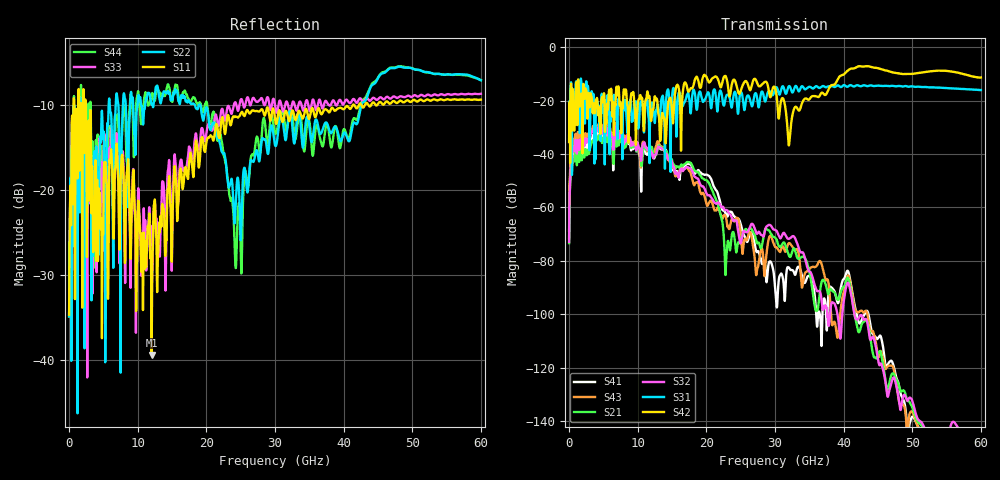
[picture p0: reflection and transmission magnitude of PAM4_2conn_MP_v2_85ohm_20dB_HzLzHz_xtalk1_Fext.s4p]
! Info: Touchstone file created by Circ.  Input file=FAB50GbE_2conn_Midplane_Examax_Topo2_v2_85ohm_20dB_HzLzHz.circ
# Hz S RI R 50
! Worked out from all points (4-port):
!   6000 points, 10 MHz to 60 GHz, reference 50 ohm
!   strongest paths, dB at 10 MHz, 15.01 GHz, 30.01 GHz, 45.01 GHz, 60 GHz:
!     S42: -35.5, -24.0, -15.3, -7.9, -11.4
!     S31: -35.4, -18.5, -15.8, -14.4, -16.1
!     S32: -72.9, -43.2, -68.4, -116.9, -151.1
!     S21: -73.4, -42.3, -71.3, -115.0, -146.2
!     S43: -71.5, -44.6, -74.7, -115.5, -158.6
!     S41: -68.7, -43.4, -90.3, -109.0, -158.7
!   lowest |S11| = -39.5 dB at 12.03 GHz (marker M1), VSWR 1.02, Z = 50.8 + j0.663 ohm
!   |S11| at or under -10 dB: start of sweep to 664.7 MHz; 2.422 GHz to 41.34 GHz (38.91 GHz wide, 178 % of centre); 41.56 GHz to 42.2 GHz (636.6 MHz wide, 1.52 % of centre)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
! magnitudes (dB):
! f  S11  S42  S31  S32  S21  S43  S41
! 10 MHz  -34.7  -35.5  -35.4  -72.9  -73.4  -71.5  -68.7
! 1.14 GHz  -12.1  -15.5  -16.6  -39.9  -44.2  -36.3  -39.1
! 12.03 GHz  -39.5  -26.6  -21.3  -39.5  -37.3  -38.4  -38.7
! 22.88 GHz  -12.5  -11.2  -18.5  -60.9  -80.2  -63.9  -62.3
! 32.06 GHz  -11.9  -36.5  -14.6  -71.8  -78.2  -73.4  -82.6
! 42.09 GHz  -10.2  -7.2  -14.3  -101.9  -106.1  -99.4  -102.0
! 60 GHz  -9.4  -11.4  -16.1  -151.1  -146.2  -158.6  -158.7
